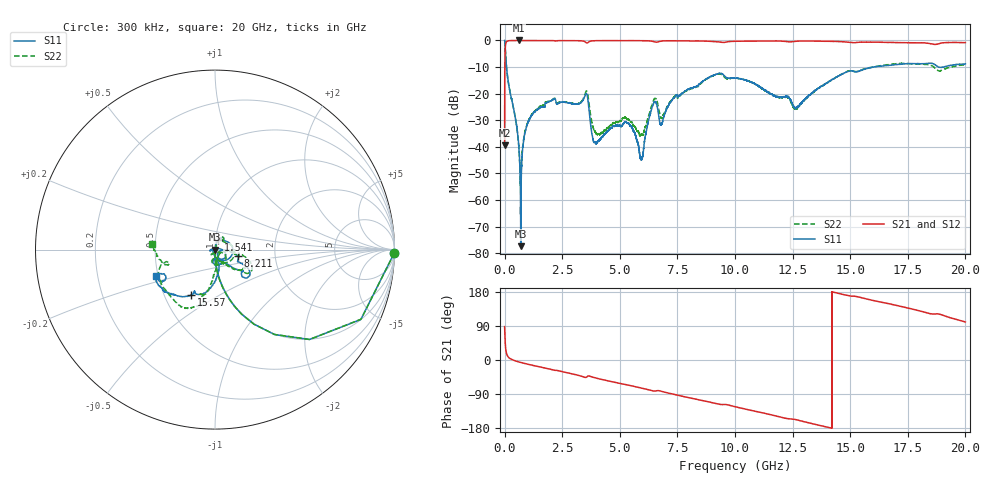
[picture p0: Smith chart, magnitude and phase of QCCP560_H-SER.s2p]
!{QCCP560}
!Johanson Technology Inc.
!www.johansontechnology.com
!Test Board Conditions:
!Substrate Type  RO4350B
!Substrate Thickness  20 mil
!Substrate Dk  3.66
!TL Type: GCPW
!TL Trace Width  36 mil
!TL Gap  12 mil
!Electrode orientation  Horizontal
!DUT TOPOLOGY	SERIES
!Mounting Pad LxW  26x36 mil
! Created Sat Jan  9 18:39:15 2021
# hz S ma R 50
! 2 Port Network Data from SP1.SP block
! freq  magS11  angS11  magS21  angS21  magS12  angS12  magS22  angS22
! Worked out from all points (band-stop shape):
!   20001 points, 300 kHz to 20 GHz, reference 50 ohm
!   highest |S21| = -0.01 dB at 640.3 MHz (marker M1); lowest = -39.4 dB at 300 kHz (marker M2)
!   |S21| within 3 dB of the highest: 28 MHz to end of sweep
!   lowest |S11| = -77.4 dB at 700.3 MHz (marker M3), VSWR 1.00, Z = 50 - j0.0011 ohm
!   |S11| at or under -10 dB: 82.47 MHz to 16.01 GHz (15.93 GHz wide, 198 % of centre); 16.02001 GHz to 16.02062 GHz (611.7 kHz wide, 0.00382 % of centre); 18.83 GHz to 19.03 GHz (192 MHz wide, 1.01 % of centre)
!   |S22| runs from -54.6 to 0.0 dB; largest |S21 - S12| = 0.016
!   S11 on the Smith chart (normalised r, x): 300 kHz: open; 1.541 GHz: 1.03, +0.11; 8.211 GHz: 1.29, -0.09; 15.57 GHz: 0.68, -0.37; 20 GHz: 0.49, -0.16
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300000  0.9993 -1.0  0.01075 88.0  0.0109 89.0  0.9999 -1.0
1.153e8  0.2298 -77.4  0.9717 12.2  0.9712 12.1  0.2304 -77.5
5.153e8  0.02599 -91.9  0.9977 -3.2  0.9971 -3.2  0.02582 -89.4
6.403e8  0.007114 -93.2  0.9986 -5.5  0.998 -5.5  0.006994 -80.4
7.003e8  0.000135 -4.7  0.998 -6.5  0.9979 -6.5  0.002098 5.3
9.803e8  0.02595 80.1  0.997 -10.7  0.9974 -10.7  0.02714 73.1
1.5413e9  0.05463 73.1  0.9945 -18.4  0.9947 -18.4  0.05737 68.2
3.3343e9  0.06901 45.8  0.9834 -42.8  0.983 -42.8  0.07059 34.4
3.5693e9  0.0977 -21.4  0.8954 -44.5  0.8955 -44.5  0.1112 -25.4
3.9233e9  0.01224 -162.5  0.9882 -47.0  0.9884 -47.0  0.01926 -85.6
5.2993e9  0.02823 -171.0  0.9912 -65.4  0.9908 -65.4  0.03371 -127.0
5.9313e9  0.005719 103.6  0.9897 -73.9  0.9914 -73.9  0.01682 -78.9
6.4293e9  0.05941 -16.7  0.9606 -81.4  0.9616 -81.4  0.06682 -30.3
6.6673e9  0.04477 -69.0  0.9468 -80.9  0.9454 -80.8  0.05748 -70.9
6.8133e9  0.02651 -27.5  0.9753 -82.8  0.9752 -82.7  0.0344 -43.0
8.2113e9  0.1314 -15.5  0.9787 -102.2  0.9772 -101.9  0.1301 -15.0
1.00003e10  0.1961 -37.1  0.9657 -123.2  0.9648 -123.2  0.1955 -32.4
1.26173e10  0.0532 -90.8  0.9621 -157.0  0.9657 -157.0  0.05102 -94.8
1.33343e10  0.1029 -78.0  0.9747 -167.7  0.9769 -167.7  0.1023 -85.6
1.55683e10  0.2839 -117.7  0.9315 163.2  0.936 162.9  0.2889 -102.0
1.66673e10  0.3374 -132.4  0.9202 148.6  0.9094 148.4  0.3518 -112.8
2e10  0.3605 -155.9  0.9095 100.4  0.8991 100.2  0.3565 175.0
